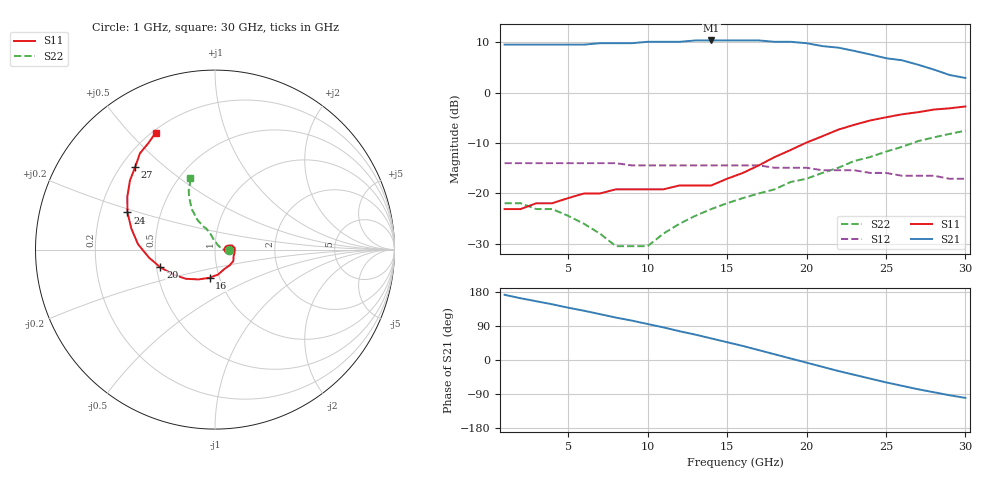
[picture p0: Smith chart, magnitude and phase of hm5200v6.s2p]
! HMMC-5200
!  S-PARAMETERS at  Vcc = 6.0V;  Rout = 100 Ohm;  Lin/out = 170pH
# GHZ  S  MA  R  50
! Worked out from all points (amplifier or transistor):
!   30 points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, 1 GHz to 30 GHz, reference 50 ohm
!   highest |S21| = 10.4 dB at 14 GHz (marker M1)
!   |S21| within 3 dB of that: start of sweep to 24.31 GHz
!   unconditionally stable (mu >= 1): start of sweep to 22 GHz
!   at 6 GHz: K = 1.12, MAG = 9.6 dB, |S12| = -14.0 dB
!   at 16 GHz: K = 1.07, MAG = 10.8 dB, |S12| = -14.4 dB
!   at 30 GHz: K = 0.89, MSG = 10.0 dB, |S12| = -17.1 dB
!   S11 on the Smith chart (normalised r, x): 1 GHz: 1.15, +0.01; 16 GHz: 0.90, -0.29; 20 GHz: 0.52, -0.12; 24 GHz: 0.32, +0.18; 27 GHz: 0.26, +0.40; 30 GHz: 0.21, +0.59
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1  0.07 4.0  3 172.0  0.2 -3.0  0.08 -1.0
2  0.07 10.0  3 163.0  0.2 -6.0  0.08 -2.0
4  0.08 15.0  3 147.0  0.2 -11.0  0.07 -4.0
6  0.1 13.0  3 130.0  0.2 -17.0  0.05 -1.0
7  0.1 10.0  3.1 121.0  0.2 -20.0  0.04 4.0
8  0.11 5.0  3.1 112.0  0.2 -23.0  0.03 15.0
10  0.11 -9.0  3.2 95.0  0.19 -28.0  0.03 61.0
11  0.11 -19.0  3.2 86.0  0.19 -31.0  0.04 81.0
13  0.12 -47.0  3.3 67.0  0.19 -37.0  0.06 99.0
14  0.12 -64.0  3.3 57.0  0.19 -40.0  0.07 102.0
16  0.16 -101.0  3.3 37.0  0.19 -47.0  0.09 106.0
17  0.19 -119.0  3.3 26.0  0.19 -50.0  0.1 108.0
18  0.23 -135.0  3.2 15.0  0.18 -53.0  0.11 110.0
19  0.27 -149.0  3.2 4.0  0.18 -56.0  0.13 113.0
20  0.32 -162.0  3.1 -7.0  0.18 -59.0  0.14 116.0
21  0.37 -173.0  2.9 -18.0  0.17 -63.0  0.16 118.0
22  0.43 176.0  2.8 -29.0  0.17 -66.0  0.18 120.0
24  0.53 157.0  2.4 -49.0  0.16 -71.0  0.23 120.0
26  0.61 141.0  2.1 -68.0  0.15 -76.0  0.29 118.0
27  0.64 134.0  1.9 -77.0  0.15 -79.0  0.33 116.0
29  0.7 122.0  1.5 -93.0  0.14 -83.0  0.39 111.0
30  0.73 117.0  1.4 -100.0  0.14 -85.0  0.42 109.0
